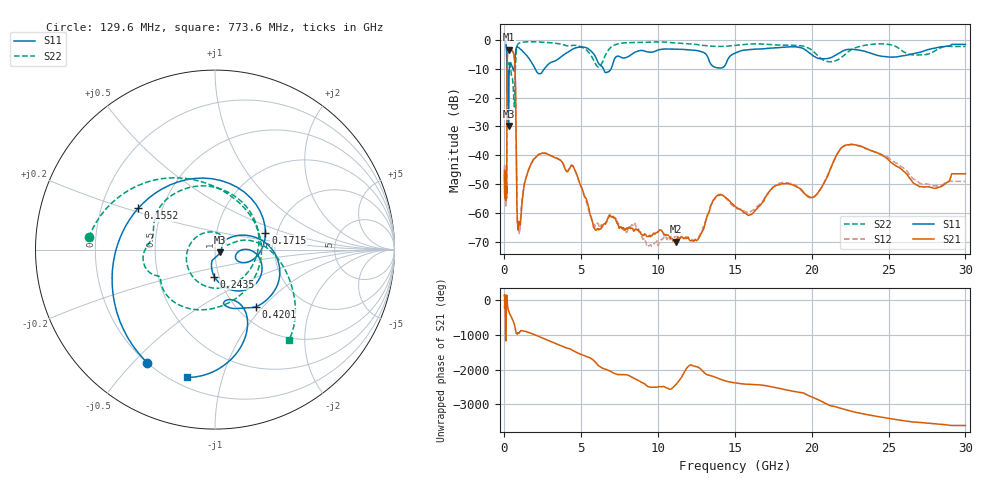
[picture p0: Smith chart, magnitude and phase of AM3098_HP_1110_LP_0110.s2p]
! Date/Time: Thu, Feb 28, 2019 8:46 AM
! Network Analyzer: Agilent Technologies E8364B Rev: A.07.50.67
! Sweep from 0.010 to 30.000 GHz, 1601 Points, Sweep Type: LOG
! Power Supply: 5.022 V, 0.002 A
# Hz S DB R 50
!freq MagS11 AngS11 MagS21 AngS21 MagS12 AngS12 MagS22 AngS22
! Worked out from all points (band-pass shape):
!   1601 points, 10 MHz to 30 GHz, reference 50 ohm
!   highest |S21| = -3.46 dB at 285.8 MHz (marker M1); lowest = -69.8 dB at 11.14 GHz (marker M2)
!   |S21| within 3 dB of the highest: 183.3 MHz to 645.7 MHz (462.4 MHz wide, 112 % of centre)
!   lowest |S11| = -29.8 dB at 263.8 MHz (marker M3), VSWR 1.07, Z = 52.9 - j1.53 ohm
!   |S11| at or under -10 dB: 170.1 MHz to 318.5 MHz (148.4 MHz wide, 60.8 % of centre); 1.993 GHz to 2.6 GHz (607.3 MHz wide, 26.4 % of centre); 6.432 GHz to 6.949 GHz (516.5 MHz wide, 7.72 % of centre)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
!   |S22| runs from -23.2 to -0.6 dB; largest |S21 - S12| = 0.0099
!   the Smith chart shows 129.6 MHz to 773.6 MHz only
!   S11 on the Smith chart (normalised r, x): 129.6 MHz: 0.20, -0.55; 155.2 MHz: 0.37, +0.22; 171.5 MHz: 1.74, +0.35; 243.5 MHz: 0.95, -0.29; 420.1 MHz: 1.21, -0.91; 773.6 MHz: 0.26, -0.77
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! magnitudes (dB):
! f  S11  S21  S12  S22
! 10 MHz  -0.4  -46.7  -43.6  -0.6
! 38.04 MHz  -0.3  -51.7  -50.6  -0.7
! 129.6 MHz  -2.7  -51.2  -53.7  -3.0
! 144.7 MHz  -4.3  -51.2  -51.2  -5.7
! 155.2 MHz  -6.3  -34.4  -34.5  -10.6
! 171.5 MHz  -10.6  -11.5  -11.5  -8.8
! 243.5 MHz  -16.5  -3.7  -3.7  -8.5
! 263.8 MHz  -29.8  -3.5  -3.5  -9.0
! 285.8 MHz  -16.4  -3.5  -3.4  -8.9
! 420.1 MHz  -8.2  -3.5  -3.5  -10.6
! 550.5 MHz  -10.1  -4.2  -4.2  -15.0
! 689.5 MHz  -6.5  -10.4  -10.4  -14.6
! 773.6 MHz  -2.8  -40.9  -40.4  -3.7
! 842.3 MHz  -2.4  -63.4  -63.3  -1.9
! 949.8 MHz  -2.8  -62.8  -66.4  -1.2
! 2.084 GHz  -10.9  -40.4  -40.4  -0.8
! 4.436 GHz  -3.3  -43.6  -43.5  -2.0
! 7.926 GHz  -6.2  -65.4  -66.5  -1.1
! 11.14 GHz  -3.3  -69.8  -67.9  -1.1
! 20.1 GHz  -5.6  -54.5  -54.4  -4.0
! 22.67 GHz  -3.4  -36.2  -36.3  -3.2
! 30 GHz  -1.6  -46.3  -49.0  -2.4
